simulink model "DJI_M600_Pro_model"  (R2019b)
settings: Solver=FixedStepAuto  StartTime=0.0  StopTime=stop_time  FixedStep=ts_hexacopter  RelTol=1e-3
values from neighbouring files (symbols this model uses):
  Alt_den = [0.1 1 0]    [Model_3D_init.m]
  Alt_err = 0.3817    [Model_3D_init.m]
  Alt_num = -[2 1]*18    [Model_3D_init.m]
  DvD = -5    [Model_3D_init.m]
  DvN = -17    [Model_3D_init.m]
  DvT = -17    [Model_3D_init.m]
  flightctrl_flag = bin2dec([HorizontalLogic; VerticalLogic; YawLogic; HorizontalCoordinate; StableMode]')    [User_defined_3D_init_run.m]
  Pden = [0.01 1]    [Model_3D_init.m]
  PI = -0.03    [Model_3D_init.m]
  pitch_max = 25/180*pi    (= 0.436332312999)    [Model_3D_init.m]
  Pnum = 100*[0.25 5]    [Model_3D_init.m]
  PP = -0.07    [Model_3D_init.m]
  r_max = 2.618    [Model_3D_init.m]
  r_min = -2.618    [Model_3D_init.m]
  Rden = [0.01 1]    [Model_3D_init.m]
  RI = 0.03    [Model_3D_init.m]
  Rnum = 100*[0.32 5]    [Model_3D_init.m]
  roll_max = 25/180*pi    (= 0.436332312999)    [Model_3D_init.m]
  RP = 0.07    [Model_3D_init.m]
  ts_hexacopter = 0.005    [Model_3D_init.m]
  UvD = 5    [Model_3D_init.m]
  UvN = 17    [Model_3D_init.m]
  UvT = 17    [Model_3D_init.m]
  Xtype = 3    [User_defined_3D_init_run.m]
  Yaw_den = [ET 1 0]    [Model_3D_init.m]
  Yaw_num = Eg*[1 Ez]    [Model_3D_init.m]
  YAWtype = 1    [User_defined_3D_init_run.m]
  Ytype = 1    [User_defined_3D_init_run.m]
  Ztype = 1    [User_defined_3D_init_run.m]
undefined symbols (not defined in the file or in its folder): DiscIntNeverNeededParam, params, Xdoublet, Xstep, YAWdoublet, YAWstep, Ydoublet, Ystep, Zdoublet, Zstep
libraries: simulink x1
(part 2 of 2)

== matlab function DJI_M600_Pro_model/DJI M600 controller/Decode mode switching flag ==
function switch_signals = decode_flag(flag_dec)
% Decode the binary mode selection flag
% Integer flag based on DJI OSDK's flightCtrl function by commenting modes in/out
%For more ref see: https://developer.dji.com/onboard-api-reference/structDJI_1_1OSDK_1_1Control_1_1CtrlData.html#a5f683c6c69478dc720245c9c2b79cf5e
%
% Construction rules and meaning
% HorizontalCoordinate = dec2bin([0 0]);   % Ground/Earth (North East position / velocity reference)
% HorizontalCoordinate = dec2bin([0 1]);    % Body (Tangential Normal position / velocity reference)
%
% HorizontalLogic = dec2bin([0 0]);         % Pitch and roll angle [deg]
% HorizontalLogic = dec2bin([0 1]);         % Horizontal velocities [m/s]
% HorizontalLogic = dec2bin([1 0]);         % Horizontal positions [m]
% HorizontalLogic = dec2bin([1 1]);         % Pitch and roll angular rate NOT IMPLEMENTED
%
% VerticalLogic = dec2bin([0 0]);            % Velocity [m/s]
% VerticalLogic = dec2bin([0 1]);            % Altitude [m]
% VerticalLogic = dec2bin([1 0]);            % Thrust [%] NOT IMPLEMENTED
%
% YawLogic = dec2bin(0);                      % Angle [deg]
% YawLogic = dec2bin(1);                      % Angular rate [deg/s]

% StableMode = dec2bin(0);                   % Drone will not keep position
                                            %when velocity command is 0 NOT IMPLEMENTED
% StableMode = dec2bin(1);                    % Drone will keep position when velocity command is 0
%
% INPUT:
% mode selection flag
% OUTPUTS:
% y(1):     HorizontalLogic
% y(2):     VerticalLogic
% y(3):     YawLogic
% y(4):     HorizontalCoordinate
%
% Institute for Computer Science and Control,  Budapest, Hungary
% Systems and Control Laboratory 2023.
% v3.0 12. June 2023.
%

flag_bin = dec2bin(flag_dec, 8); % Convert decimal value to 8 bits binary

% Extract the separate flags
HorizontalLogicSwitch = bin2dec(flag_bin(1:2));

VerticalLogicSwitch = bin2dec(flag_bin(3:4));

YawLogicSwitch = bin2dec(flag_bin(5));

HorizontalCoordinateSwitch = bin2dec(flag_bin(6:7));

switch_signals = [HorizontalLogicSwitch, VerticalLogicSwitch, YawLogicSwitch, HorizontalCoordinateSwitch];

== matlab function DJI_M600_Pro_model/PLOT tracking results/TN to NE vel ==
function y = fcn(u)
% Transform Tangential-Normal to North-East
% Inputs
% u(1):     Tangential position / velocity
% u(2):     Normal position / velocity
% u(3):     Real yaw angle
% Outputs
% N:    North position / velocity
% E:    East position / velocity
%
% Institute for Computer Science and Control, Budapest, Hungary
% Systems and Control Laboratory 2023.
% v3.0 12. June 2023.

y = [u(1)*cos(u(3))-u(2)*sin(u(3)); u(1)*sin(u(3))+u(2)*cos(u(3))];

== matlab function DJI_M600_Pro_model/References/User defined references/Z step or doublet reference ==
function y = fcn(u, Zstep, Zdoublet)
% Z direction reference signal generation
% Inputs:
% u(1): type of required reference
% u(2): absolute time [s]
% Parameters:
% Zstep:    parameter structure of step (type 1) reference
% Zdoublet: parameter  structures of doublet (type 2), half doublet (type 3) and
%           elonged doublet (type 4) references
% For details see: User_defined_3D_init_run.m script
%
% Institute for Computer Science and Control,  Budapest, Hungary
% Systems and Control Laboratory 2023.
% v3.0 12. June 2023.
% 


    persistent start    
    % Save parameter structures into local values:
    step=Zstep;
    doublet=Zdoublet;
    
    % Initialize persistent variable upon startup
    if isempty(start)
        start = 0;
    end
    
    % Save time of start
    if (start==0)
        start = u(2);
    end
    
    % Default value for case of undefined parameters:
    ref=0;
    
    switch u(1)
        case 1 % step reference required
            if (u(2)<start + step.step) % Output before step
                ref=step.zero;
            else                        % Output after step
                ref=step.zero + step.amp;
            end   
            
        case 2 % doublet reference required
            if (u(2)<start + doublet.step) % Output before doublet
                ref=doublet.zero;
            elseif (u(2)>=(start + doublet.step) && u(2)<(start + doublet.step + doublet.period/2)) % First, positive period
                ref=doublet.zero + doublet.amp;
            elseif (u(2)>=(start + doublet.step + doublet.period/2) && u(2)<(start + doublet.step + doublet.period)) % Second, negative period
                ref=doublet.zero- doublet.amp;
            else                            % Output after doublet
                ref=doublet.zero;
            end                    
        case 3 % half doublet reference required
            if (u(2)<start + doublet.step) % Output before half doublet
                ref=doublet.zero;
            elseif (u(2)>=(start + doublet.step) && u(2)<(start + doublet.step + doublet.period)) % Half doublet output (positive)
                ref=doublet.zero + doublet.amp;            
            else                           % Output after half doublet
                ref=doublet.zero; 
            end   
        case 4 % elongated doublet reference required (1.5 period long with gap)
            if (u(2)<start + doublet.step)      % Output before elongated doublet
                ref=doublet.zero;
            elseif (u(2)>=(start + doublet.step) && u(2)<(start + doublet.step + doublet.period/2)) % First, positive period
                ref=doublet.zero + doublet.amp;
            elseif (u(2)>=(start + doublet.step + doublet.period/2) && u(2)<(start + doublet.step + doublet.period)) % Gap with zero level output
                ref=doublet.zero;
            elseif (u(2)>=(start + doublet.step + doublet.period) && u(2)<(start + doublet.step + 3*doublet.period/2)) % Second, negative period
                ref=doublet.zero - doublet.amp;
            else                                % Output after elongated doublet
                ref=doublet.zero;
            end
    end
    
    y = ref; % Function output (actual value of reference)
end

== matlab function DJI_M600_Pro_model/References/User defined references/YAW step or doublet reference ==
function y = fcn(u, YAWstep, YAWdoublet)
% YAW reference signal generation
% Inputs:
% u(1): type of required reference
% u(2): absolute time [s]
% Parameters:
% YAWstep:    parameter structure of step (type 1) reference
% YAWdoublet: parameter  structures of doublet (type 2), half doublet (type 3) and
%             elonged doublet (type 4) references
% For details see: User_defined_3D_init_run.m script
%
% Institute for Computer Science and Control,  Budapest, Hungary
% Systems and Control Laboratory 2023.
% v3.0 12. June 2023.
% 


    persistent start    
    % Save parameter structures into local values:
    step=YAWstep;
    doublet=YAWdoublet;
    
    % Initialize persistent variable upon startup
    if isempty(start)
        start = 0;
    end
    
    % Save time of start
    if (start==0)
        start = u(2);
    end
    
    % Default value for case of undefined parameters:
    ref=0;
    
    switch u(1)
        case 1 % step reference required
            if (u(2)<start + step.step) % Output before step
                ref=step.zero;
            else                        % Output after step
                ref=step.zero + step.amp;
            end   
            
        case 2 % doublet reference required
            if (u(2)<start + doublet.step) % Output before doublet
                ref=doublet.zero;
            elseif (u(2)>=(start + doublet.step) && u(2)<(start + doublet.step + doublet.period/2)) % First, positive period
                ref=doublet.zero + doublet.amp;
            elseif (u(2)>=(start + doublet.step + doublet.period/2) && u(2)<(start + doublet.step + doublet.period)) % Second, negative period
                ref=doublet.zero- doublet.amp;
            else                            % Output after doublet
                ref=doublet.zero;
            end                    
        case 3 % half doublet reference required
            if (u(2)<start + doublet.step) % Output before half doublet
                ref=doublet.zero;
            elseif (u(2)>=(start + doublet.step) && u(2)<(start + doublet.step + doublet.period)) % Half doublet output (positive)
                ref=doublet.zero + doublet.amp;            
            else                           % Output after half doublet
                ref=doublet.zero; 
            end   
        case 4 % elongated doublet reference required (1.5 period long with gap)
            if (u(2)<start + doublet.step)      % Output before elongated doublet
                ref=doublet.zero;
            elseif (u(2)>=(start + doublet.step) && u(2)<(start + doublet.step + doublet.period/2)) % First, positive period
                ref=doublet.zero + doublet.amp;
            elseif (u(2)>=(start + doublet.step + doublet.period/2) && u(2)<(start + doublet.step + doublet.period)) % Gap with zero level output
                ref=doublet.zero;
            elseif (u(2)>=(start + doublet.step + doublet.period) && u(2)<(start + doublet.step + 3*doublet.period/2)) % Second, negative period
                ref=doublet.zero - doublet.amp;
            else                                % Output after elongated doublet
                ref=doublet.zero;
            end
    end
    
    y = ref; % Function output (actual value of reference)
end

== matlab function DJI_M600_Pro_model/DJI M600 controller/Yaw angle error handling
PI ctrl with AW ==
function r_ref = fcn(psi_ref,psi,P_yaw)
% P control of yaw angle
% Inputs:
% psi_ref:  yaw angle reference
% psi:      yaw angle 
% Parameter:
% P_yaw:    proportional gain
% Output:   
% r_ref:    yawrate reference
%
% Institute for Computer Science and Control,  Budapest, Hungary
% Systems and Control Laboratory 2023.
% v3.0 12. June 2023.
%  

% Convert error due to change between +/-180 degs to prevent latent large
% angular errors
err=psi_ref-psi;
if err>185/180*pi
    err=psi_ref-(2*pi+psi);
end
if err<-185/180*pi
    err=2*pi+psi_ref-psi;
end
   
% Proportional control
r_ref=P_yaw*err;

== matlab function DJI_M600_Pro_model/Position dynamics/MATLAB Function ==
function y_B = inertialtobody(u)
% Transformation of earth gravitational acceleration vector into body system
% Inputs:
% u(1:3):   Earth gravity vector [m/s^2]
% u(4:6):   roll, pitch, yaw Euler angles [rad]
%
% Institute for Computer Science and Control,  Budapest, Hungary
% Systems and Control Laboratory 2023.
% v3.0 12. June 2023.
%

% Separate inputs
% Earth gravity vector
u_I = u(1:3);
% Euler angles
phi = u(4);
theta = u(5);
psi = u(6);

% Create inertial to body rotation matrix
R_1 = [1 0 0; 0 cos(phi) sin(phi); 0 -sin(phi) cos(phi)];
R_2 = [cos(theta) 0 -sin(theta); 0 1 0; sin(theta) 0 cos(theta)];
R_3 = [cos(psi) sin(psi) 0; -sin(psi) cos(psi) 0; 0 0 1];

R_BI = R_1*R_2*R_3;

% Output is body gravitational acceleration vector
y_B = R_BI*u_I;

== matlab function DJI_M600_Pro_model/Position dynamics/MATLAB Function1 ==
function v_I = v_bodytoinertial(u)
% Transformation of input body aircraft velocity into inertial velocity
% Inputs:
% u(1:3):   Rigid body velocity [m/s]
% u(4:6):   roll, pitch, yaw Euler angles [rad]
%
% Institute for Computer Science and Control,  Budapest, Hungary
% Systems and Control Laboratory 2023.
% v3.0 12. June 2023.
%

% Separate inputs
% body velocity
v_B = [u(1); u(2); u(3)];
% Euler angles
phi = u(4);
theta = u(5);
psi = u(6);

% Create body to inertial rotation matrix
R_1 = [1 0 0; 0 cos(phi) -sin(phi); 0 sin(phi) cos(phi)];
R_2 = [cos(theta) 0 sin(theta); 0 1 0; -sin(theta) 0 cos(theta)];
R_3 = [cos(psi) -sin(psi) 0; sin(psi) cos(psi) 0; 0 0 1];

R_IB = R_3*R_2*R_1;

% Output is inertial velocity
v_I = R_IB*v_B;

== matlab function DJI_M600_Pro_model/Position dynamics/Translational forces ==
function y = fcn(u,params)
% Function to calculate body translational forces
%
% Institute for Computer Science and Control,  Budapest, Hungary
% Systems and Control Laboratory 2023.
% v3.0 12. June 2023.
%
% Inputs:
% u(1)-u(6):    rotor angular rates [rad/s]
% u(7)-u(9):    Airspeed in body system [m/s]
% Outputs:
% Fx X body force [N]
% Fy Y body force [N]
% Fz Z body force [N]

% Vertical gain:
Kc=0.0243*u(9).^2+2.8851;

% Air geometric constant
cAG=params.rho*params.A*params.R;

% Body Z force
Fz=-params.cT0*cAG*params.R*sum(u(1:6).^2)-Kc/100*cAG*u(9)*sum(u(1:6));

% Body X force
Fx=-params.Khx*cAG*u(7)*sum(u(1:6))/100-params.Kx*u(7)*abs(u(7));

% Body Y force
Fy=-params.Khy*cAG*u(8)*sum(u(1:6))/100-params.Ky*u(8)*abs(u(8));

y = [Fx; Fy; Fz];

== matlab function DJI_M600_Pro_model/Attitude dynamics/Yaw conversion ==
function y = fcn(u)
% Conversion of yaw angle between +/-pi
%
% Institute for Computer Science and Control,  Budapest, Hungary
% Systems and Control Laboratory 2023.
% v3.0 12. June 2023.
%

y1=mod(u,2*pi);
if y1>pi
    y=y1-2*pi;
else
    y = y1;
end

== matlab function DJI_M600_Pro_model/DJI M600 controller/Tangential // normal 
HORIZ references ==
function y  = TNctrl(t,X_ref,Y_ref,HorizLogic)
% Processing of references for control in Tangential / Horizontal
% directions (aligned with body system of M600)
% Inputs:
% t:            time [s]
% X_ref:        X reference
% Y_ref:        Y reference
% HorizLogic:   horizontal logic flag
% Outputs:
% v_T_ref:      Tangential velocity reference
% v_N_ref:      Normal velocity reference
% Phi_ref:      Roll reference
% Theta_ref:    Theta reference
% HLogic:       the same flight mode flag as the input, or a modified one
%               when returning from angle track to braking mode with zero
%               velocity
% X_ref:        X position reference (North / Tangential)
% Y_ref:        Y position reference (East / Normal)
%
% Institute for Computer Science and Control,  Budapest, Hungary
% Systems and Control Laboratory 2023.
% v3.0 12. June 2023.
%

% Persistent variables:
% Init flag of Position kick control
persistent Pinit
% Start time of position kick control
persistent t0
% X and Y reference amplitudes to be applied
% (not necessarily the same as X_ref and Y_ref)
persistent Xamp
persistent Yamp
% Flag for Position step mode
persistent Pstep

% Initialize permanent variables upon startup
if isempty(Pinit)
    Pinit=0;
    t0=0;
    Xamp=0;
    Yamp=0;
    Pstep=0;
end

% Switch horizontal logic flag
switch HorizLogic
    case 0 % Angle references
        if (X_ref~=0 || Y_ref~=0)  % Normal angle tracking (convert deg to rad)   
            y=[0; 0; X_ref/180*pi; Y_ref/180*pi; 0; 0; 0];
        elseif (X_ref==0 && Y_ref==0) % Change to velocity track for braking
            y=[0; 0; 0; 0; 1; 0; 0];
        else    % Safe output with zero references
            y=[0; 0; 0; 0; 1; 0; 0];
        end
    case 1 % Velocity references
        % Give out X and Y references as velocities
        y=[X_ref; Y_ref; 0; 0; 1; 0; 0];
    case 2 % Position references
        if (X_ref~=0 || Y_ref~=0 || 1==Pinit) % Nonzero references start kick control
            if (0==Pinit)
                Pinit=1;
                t0=t;
                Xamp=X_ref;
                Yamp=Y_ref;
            end
            if (t-t0<=0.75 && 0==Pstep) % Not real position, limited time velocity reference is given (kick control)
                if (t-t0>0.5 && (X_ref~=0 || Y_ref~=0)) % Switch to step reference mode if long reference comes
                    Pstep=1;
                end
                y=[Xamp; Yamp; 0; 0; 1; X_ref; Y_ref];
            elseif (1==Pstep) % Position step mode with long reference
                y=[sign(X_ref)*min([abs(X_ref)/2,3]); sign(Y_ref)*min([abs(Y_ref)/2,3]); 0; 0; 1; X_ref; Y_ref];
                % Switch back from position step mode if references are
                % again zero
                if (0==X_ref && 0==Y_ref)
                    Pstep=0;
                end
            else % Safe output with zero references, and re-init position kick mode
                y=[0; 0; 0; 0; 1; 0; 0];
                Pinit=0;                
            end
        else % Safe output with zero references
            y=[0; 0; 0; 0; 1; 0; 0];
        end            
    otherwise   % Safe mode with velocity flag and zero velocity references
        y=[0; 0; 0; 0; 1; 0; 0];
end
